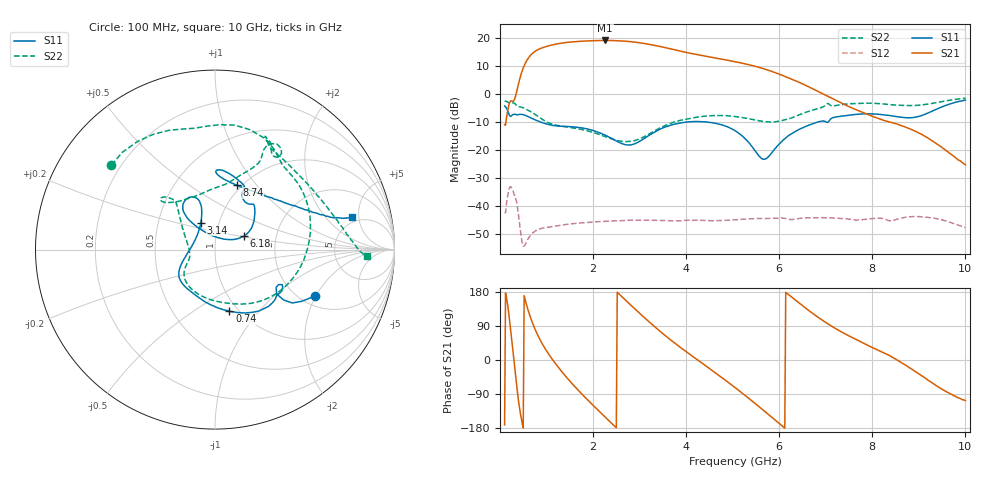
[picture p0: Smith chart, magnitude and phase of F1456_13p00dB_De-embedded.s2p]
! Integrated Device Technology
! Corporate Headquarters
! 6024 Silver Creek Valley Road
! San Jose, CA 95138  USA
! Phone:  1-408-284-8200
! Toll Free:  1-800-223-1366
! Webpage:  http://www.idt.com/
! Timing and RF Division
! 515 Groton Road, Suite 102
! Westford, MA 01886-6024
! Device:  F1456
! Description: 6-bit 0.5 dB Transmit Variable Gain Amplifier
! Frequency:  2100.0 -  2950.00 MHz
! Package:  6x6 mm Thin QFN Plastic Package: 28 pin
! State:  26
! Atten State:  13.0 dB
! Voltage:  +5.00 Volts
! Current:  217.017 mA
! Data:  The device was measured on a the F1455 evaluation board which has
!  individual transmission lines to the RF pins.  Data was collected
!  using a calibrated network analyzer.  The evaluation board was
!  de-embedded using a TRL calibration technique.
!  The reference plane is the edge of the package pin.
!  Pin  1 = CSb
!  Pin  2 = DATA
!  Pin  3 = CLK
!  Pin  4 = RSET
!  Pin  5 = GND
!  Pin  6 = RFIN  = Port 1
!  Pin  7 = GND
!  Pin  8 = NC
!  Pin  9 = NC
!  Pin 10 = NC
!  Pin 11 = NC
!  Pin 12 = NC
!  Pin 13 = NC
!  Pin 14 = /STBY
!  Pin 15 = GND
!  Pin 16 = RFOUT  = Port 2
!  Pin 17 = GND
!  Pin 18 = NC
!  Pin 19 = NC
!  Pin 20 = NC
!  Pin 21 = GND
!  Pin 22 = NC
!  Pin 23 = GND
!  Pin 24 = NC
!  Pin 25 = NC
!  Pin 26 = NC
!  Pin 27 = GND
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# GHz S dB R 50
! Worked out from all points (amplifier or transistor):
!   496 points, 100 MHz to 10 GHz, reference 50 ohm
!   highest |S21| = 19.2 dB at 2.26 GHz (marker M1)
!   |S21| within 3 dB of that: 851.6 MHz to 3.668 GHz (2.816 GHz wide, 125 % of centre)
!   unconditionally stable (mu >= 1): start of sweep to end of sweep
!   at 1.74 GHz: K = 10.09, MAG = 19.4 dB, |S12| = -46.0 dB
!   at 5.06 GHz: K = 18.62, MAG = 12.5 dB, |S12| = -44.9 dB
!   at 10 GHz: K = 243.00, MAG = -15.6 dB, |S12| = -47.7 dB
!   S11 on the Smith chart (normalised r, x): 100 MHz: 2.35, -1.96; 740 MHz: 0.91, -0.71; 3.14 GHz: 0.82, +0.25; 6.18 GHz: 1.36, +0.21; 8.74 GHz: 0.95, +0.80; 10 GHz: 4.30, +4.06
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0.1  -4.25 -25.2  -10.89 -171.2  -42.27 47.4  -2.56 140.8
0.32  -7.19 -32.3  -1.57 -20.8  -36.37 -144.4  -3.36 66.2
0.44  -7.21 -42.2  6.33 -141.7  -48.75 138.5  -4.56 38.5
0.58  -7.81 -59.2  12.12 141.9  -52.44 169.3  -5.54 5.8
0.74  -9.06 -76.8  15.14 85.2  -49.09 137.5  -7.05 -27.0
0.98  -10.54 -100.2  16.94 28.1  -47.68 92.5  -9.70 -67.8
1.2  -11.32 -116.9  17.87 -10.7  -47.15 67.6  -11.05 -94.4
1.5  -11.62 -133.7  18.59 -55.5  -46.40 42.3  -11.87 -121.2
1.76  -12.07 -143.8  18.92 -89.8  -45.97 25.0  -12.63 -136.2
2.26  -14.65 -161.7  19.18 -150.6  -45.43 -3.0  -15.17 -153.5
2.66  -17.86 167.2  18.97 162.3  -45.15 -23.2  -16.91 -169.4
3.14  -15.39 117.6  18.00 107.7  -45.01 -47.0  -14.81 156.3
3.4  -12.84 109.0  17.17 79.9  -45.10 -59.5  -12.44 141.7
3.74  -10.77 108.2  15.90 46.0  -45.28 -73.8  -9.98 131.5
4.1  -9.84 114.3  14.56 13.2  -45.11 -88.7  -8.64 130.3
5.06  -13.13 131.3  11.57 -73.6  -44.89 -130.6  -8.01 137.7
5.64  -23.16 82.7  9.21 -130.7  -44.43 -162.1  -9.71 122.1
6.18  -15.08 25.0  5.91 174.6  -44.65 164.8  -8.89 83.8
6.7  -10.69 40.9  2.09 124.6  -44.16 137.9  -5.78 64.6
8.36  -7.61 87.8  -9.87 12.4  -45.19 67.4  -3.74 62.4
8.74  -8.39 71.4  -11.98 -15.6  -43.90 58.0  -4.07 49.1
10  -2.12 13.4  -25.20 -107.1  -47.68 -24.3  -1.46 -2.6
